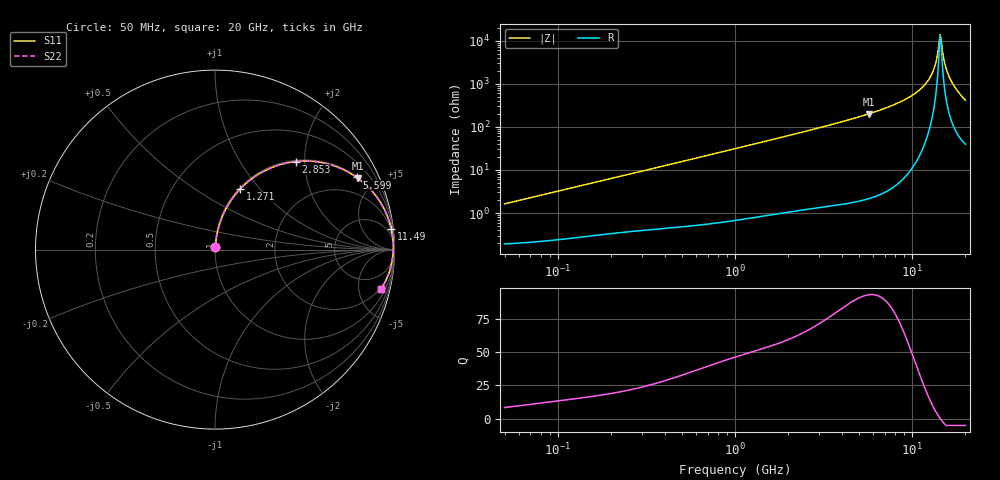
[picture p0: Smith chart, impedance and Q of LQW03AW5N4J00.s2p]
!Murata Part Number: LQW03AW5N4J00
!These Parameters are Measured in Series Mode Connection
!  o--[Z]--o
!Port1  Port2
!  o-------o
!Freq. Start=50[MHz] Stop=20[GHz], 401[Steps]
# Hz S RI R 50
!Freq.(Hz) S11(Real) S11(Imag) S21(Real) S21(Imag) S12(Real) S12(Imag) S22(Real) S22(Imag)
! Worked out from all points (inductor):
!   401 points, 50 MHz to 20 GHz, reference 50 ohm
!   read as one part in series: L = 5.15 nH near 51.52 MHz
!   highest Q = 93 at 5.683 GHz (marker M1), where L = 5.59 nH
!   self-resonance near 14.39 GHz
!   S11 on the Smith chart (normalised r, x): 50 MHz: 1.00, +0.03; 1.271 GHz: 1.02, +0.79; 2.853 GHz: 1.03, +1.81; 5.599 GHz: 1.04, +3.91; 11.49 GHz: 2, +17; 20 GHz: 1.79, -8.20
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5e7  0.00218 0.0161  0.9978 -0.0161  0.9978 -0.0161  0.00218 0.0161
1.364002e8  0.00465 0.0432  0.9954 -0.0432  0.9954 -0.0432  0.00465 0.0432
3.721004e8  0.0174 0.1138  0.9826 -0.1138  0.9826 -0.1138  0.0174 0.1138
1e9  0.093 0.2798  0.907 -0.2798  0.907 -0.2798  0.093 0.2798
1.270815e9  0.1397 0.3369  0.8603 -0.3369  0.8603 -0.3369  0.1397 0.3369
2.728004e9  0.4269 0.4873  0.5731 -0.4873  0.5731 -0.4873  0.4269 0.4873
2.853386e9  0.4499 0.4904  0.5501 -0.4904  0.5501 -0.4904  0.4499 0.4904
5.598765e9  0.7903 0.4017  0.2097 -0.4017  0.2097 -0.4017  0.7903 0.4017
5.683258e9  0.7967 0.3972  0.2033 -0.3972  0.2033 -0.3972  0.7967 0.3972
7.442007e9  0.8937 0.3024  0.1063 -0.3024  0.1063 -0.3024  0.8937 0.3024
9.600142e9  0.9555 0.1972  0.0445 -0.1972  0.0445 -0.1972  0.9555 0.1972
1.149051e10  0.982 0.1158  0.018 -0.1158  0.018 -0.1158  0.982 0.1158
1.238412e10  0.9887 0.0797  0.0113 -0.0797  0.0113 -0.0797  0.9887 0.0797
1.314879e10  0.992 0.0497  0.008 -0.0497  0.008 -0.0497  0.992 0.0497
1.354865e10  0.9929 0.0342  0.00706 -0.0342  0.00706 -0.0342  0.9929 0.0342
1.417136e10  0.9933 0.0104  0.00665 -0.0104  0.00665 -0.0104  0.9933 0.0104
1.438523e10  0.9932 0.00221  0.0068 -0.00221  0.0068 -0.00221  0.9932 0.00221
1.482269e10  0.9924 -0.0144  0.00757 0.0144  0.00757 0.0144  0.9924 -0.0144
1.550395e10  0.99 -0.0403  0.01 0.0403  0.01 0.0403  0.99 -0.0403
1.646126e10  0.9838 -0.0769  0.0162 0.0769  0.0162 0.0769  0.9838 -0.0769
1.800918e10  0.9664 -0.1373  0.0336 0.1373  0.0336 0.1373  0.9664 -0.1373
2e10  0.9257 -0.2187  0.0743 0.2187  0.0743 0.2187  0.9257 -0.2187
